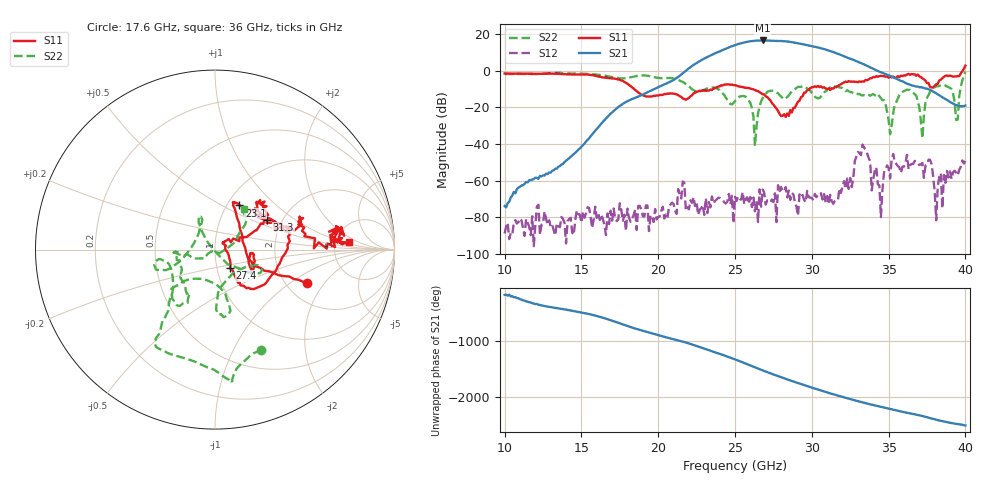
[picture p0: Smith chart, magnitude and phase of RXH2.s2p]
!Keysight Technologies,M9808A,MY58100618,A.14.70.03
!Date: Monday, February 27, 2023 13:43:07
!Correction: S11(Cdelta 2-Port  )
!S21(Cdelta 2-Port  )
!S12(Cdelta 2-Port  )
!S22(Cdelta 2-Port  )
!S2P File: Measurements: S11, S21, S12, S22:
# Hz S  RI  R 50
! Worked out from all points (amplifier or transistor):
!   301 points, 10 GHz to 40 GHz, reference 50 ohm
!   highest |S21| = 16.5 dB at 26.8 GHz (marker M1)
!   |S21| within 3 dB of that: 24.85 GHz to 29.94 GHz (5.09 GHz wide, 18.6 % of centre)
!   unconditionally stable (mu >= 1): start of sweep to 39.83 GHz
!   at 15 GHz: K = 93560.80, MAG = -32.0 dB, |S12| = -83.0 dB
!   at 25 GHz: K = 227.79, MAG = 14.8 dB, |S12| = -68.9 dB
!   at 40 GHz: K = -111.03, MSG = 15.1 dB, |S12| = -49.3 dB
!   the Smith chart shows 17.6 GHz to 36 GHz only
!   S11 on the Smith chart (normalised r, x): 17.6 GHz: 2.58, -1.37; 23.1 GHz: 1.14, +0.61; 27.4 GHz: 1.15, -0.24; 31.3 GHz: 1.67, +0.62; 36 GHz: 6.59, +1.31
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1e10  0.0339 0.8435  -0.000197 -4.51e-05  -3.29e-05 1.5e-05  0.7259 0.3723
1.5e10  0.7657 0.2148  -0.00459 -0.00706  -3.67e-05 -6.08e-05  0.6435 -0.5304
1.76e10  0.5127 -0.1857  0.0974 0.0647  0.000153 -3.58e-05  0.2571 -0.5571
2e10  0.2096 -0.0191  -0.347 -0.0722  8.15e-05 5.96e-05  -0.1126 -0.6238
2.2e10  0.1387 0.1154  0.8367 0.813  1.4e-05 0.000163  -0.2511 -0.276
2.31e10  0.1351 0.2462  1.192 -1.918  2.85e-06 -0.000334  -0.312 -0.0523
2.4e10  0.3432 0.1482  -2.644 -2.057  3.38e-06 -0.000339  -0.2746 -0.1145
2.5e10  0.4057 0.00786  -2.408 4.367  -0.000278 0.000228  -0.0831 0.1215
2.55e10  0.3398 -0.1173  2.414 5.241  -0.000462 0.000149  -0.0808 0.1889
2.6e10  0.253 -0.2043  6.26 1.113  -0.000124 0.000335  -0.075 0.1081
2.68e10  0.1373 -0.1819  1.418 -6.555  2.35e-05 -0.000573  0.1407 -0.1066
2.74e10  0.0834 -0.1029  -5.091 -4.158  6.69e-05 -0.000298  0.2592 -0.1205
2.8e10  0.0576 -0.00374  -6.071 2.256  0.000438 0.000508  0.17 -0.0966
2.86e10  0.0659 0.0525  -1.182 5.99  -0.00026 -0.000142  0.0171 -0.24
2.93e10  0.1771 0.0702  4.372 3.203  0.000212 0.00028  0.0349 -0.3613
3e10  0.2962 0.1924  4.215 -2.03  0.000103 0.000322  0.0569 -0.2417
3.06e10  0.2516 0.276  0.8169 -4.006  0.000428 -0.000132  -0.1118 -0.1619
3.13e10  0.2894 0.1651  -2.453 -2.259  0.000238 0.000134  -0.2363 -0.2762
3.27e10  0.4776 0.1535  -0.8108 1.819  -0.00109 -0.000446  -0.1759 -0.1754
3.5e10  0.635 0.0996  0.5533 -0.5013  -0.000744 0.00206  -0.0393 -0.0223
3.6e10  0.744 0.0441  -0.1228 -0.4735  0.0017 0.0017  0.1592 0.2261
4e10  1.121 -0.7989  0.1075 0.0322  -0.000847 0.00332  0.4779 -0.8217
